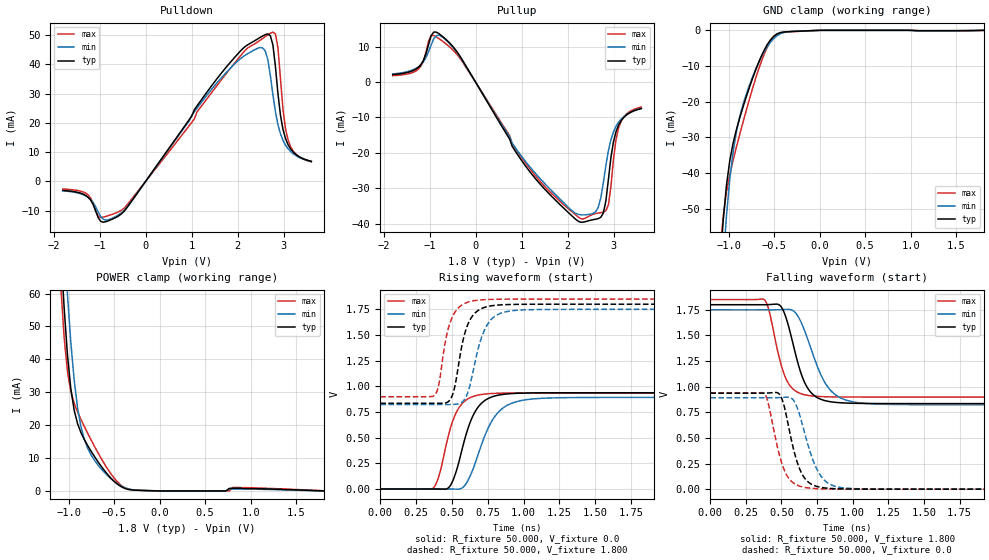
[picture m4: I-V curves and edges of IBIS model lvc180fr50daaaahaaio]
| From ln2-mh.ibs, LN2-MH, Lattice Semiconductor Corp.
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|   Model lvc180fr50daaaahaaio
[Model] lvc180fr50daaaahaaio
| Clamp models do not include dynamic input termination. Please refer to
| the lvc180axxxdaaaahaain model for input termination.
Model_type I/O
Polarity   Non-Inverting
Enable   Active-Low
Vinl =  0.630V
Vinh =  1.170V
Vmeas =  0.900V
Cref =  0.0F
Rref =  1.000M
Vref =  0.0V
C_comp   2.000pF   1.500pF   2.500pF
[Temperature Range]   25.000   0.125k   -40.000
[Voltage Range]   1.800V   1.750V   1.850V
[C Comp Corner]
C_comp   2.000pF   1.500pF   2.500pF
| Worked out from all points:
|   slope of the pulldown table from 0 to 0.27 V, typ, clamps not added: 44.9 ohm
|   slope of the pullup table from 0 to 0.27 V, typ, clamps not added: 45.5 ohm
|   GND clamp passes 1 mA (typ) near -0.47 V on its own axis
|   POWER clamp passes 1 mA (typ) near -0.40 V on its own axis
|   rising waveform, R_fixture 50.000, V_fixture 0.0: 20-80 % time 127ps typ, 160ps min, 110ps max; typ from 0 V to 0.938 V
|   rising waveform, R_fixture 50.000, V_fixture 1.800: 20-80 % time 87.8ps typ, 107ps min, 80.7ps max; typ from 0.835 V to 1.8 V
|   falling waveform, R_fixture 50.000, V_fixture 1.800: 20-80 % time 121ps typ, 162ps min, 101ps max; typ from 1.8 V to 0.835 V
|   falling waveform, R_fixture 50.000, V_fixture 0.0: 20-80 % time 102ps typ, 125ps min, 98.2ps max; typ from 0.937 V to 0 V
[Pulldown]
|Voltage   I(typ)   I(min)   I(max)
-1.8V     -3.079mA   -3.208mA   -2.604mA
-1.25V    -5.37mA    -5.445mA   -4.579mA
-975mV    -13.65mA   -11.99mA   -12.31mA
-480mV    -10.42mA   -10.07mA   -9.325mA
2.05V     44.35mA    41.79mA    42.66mA
2.545V    49.68mA    45.59mA    48.83mA
2.655V    50.36mA    41.57mA    50.03mA
2.765V    46.65mA    29.71mA    50.99mA
2.875V    29.99mA    19.42mA    45.69mA
2.93V     22.57mA    16.27mA    35.05mA
3.095V    12.53mA    11.14mA    14.19mA
3.6V      6.866mA    6.794mA    6.674mA
[Pullup]
|Voltage   I(typ)   I(min)   I(max)
-1.8V     2.133mA    2.309mA    1.821mA
-1.24V    4.215mA    4.333mA    3.727mA
-965mV    13.12mA    10.53mA    13.16mA
-745mV    13.21mA    12.97mA    11.84mA
1.125V    -24.42mA   -23.11mA   -23.58mA
2.28V     -39.63mA   -37.53mA   -38.61mA
2.665V    -38.63mA   -35.4mA    -37.04mA
2.83V     -33.63mA   -23.61mA   -36.38mA
2.885V    -27.55mA   -19.4mA    -34.71mA
2.995V    -16.89mA   -14.09mA   -21.87mA
3.105V    -12.18mA   -11.35mA   -12.99mA
3.6V      -7.446mA   -7.445mA   -7.067mA
[GND_clamp]
|Voltage   I(typ)   I(min)   I(max)
-1.8V     -571mA     -571.9mA   -573mA
-1.097V   -67.89mA   -81.9mA    -63.82mA
-1.06V    -53.86mA   -65.72mA   -52.69mA
-1.023V   -43.6mA    -52.29mA   -45.48mA
-986mV    -36.55mA   -41.78mA   -40.47mA
-949mV    -31.59mA   -33.97mA   -36.38mA
-912mV    -27.73mA   -28.25mA   -32.63mA
-838mV    -21.28mA   -20.51mA   -25.51mA
-616mV    -5.929mA   -6.39mA    -7.151mA
-468mV    -1.006mA   -1.514mA   -1.077mA
-24mV     -25.08uA   -21.99uA   -30.46uA
1.8V      -83.5nA    0A         -36.66uA
[POWER_clamp]
|Voltage   I(typ)   I(min)   I(max)
-1.789V   617.6mA    624.8mA    616.1mA
-1.086V   74.57mA    97.6mA     62.94mA
-1.049V   56.15mA    77.62mA    47.03mA
-1.012V   41.52mA    60.02mA    36.39mA
-975mV    31.15mA    45.29mA    30.27mA
-938mV    24.56mA    33.75mA    26.65mA
-901mV    20.5mA     25.36mA    24.04mA
-827mV    15.64mA    15.72mA    19.63mA
-679mV    8.958mA    7.957mA    11.71mA
-420mV    1.258mA    1.471mA    1.65mA
-13mV     8.76uA     8.311uA    10.26uA
1.8V      0A         0A         63.06uA
[Ramp]
| variable   typ   min   max
dV/dt_r   0.563/0.127n   0.536/0.160n   0.562/0.110n
dV/dt_f   0.579/0.121n   0.556/0.163n   0.571/0.101n
R_load = 50.000
[Rising Waveform]
R_fixture= 50.000
V_fixture= 0.0
V_fixture_min= 0.0
V_fixture_max= 0.0
|time   V(typ)   V(min)   V(max)
0s        2.404uV    12.25uV    1.1uV
369ps     71.87uV    58.48uV    8.909mV
411ps     -495.8uV   80.61uV    136.3mV
475ps     11.17mV    -333.7uV   519.2mV
598ps     527.8mV    50.69mV    865.8mV
666ps     763.7mV    267.7mV    909.3mV
764ps     888.9mV    626.7mV    928.9mV
914ps     929.1mV    833.7mV    935mV
1.244ns   937.1mV    888.8mV    936.2mV
10ns      937.5mV    892.5mV    936.2mV
[Rising Waveform]
R_fixture= 50.000
V_fixture= 1.800
V_fixture_min= 1.750
V_fixture_max= 1.850
|time   V(typ)   V(min)   V(max)
0s        834.8mV    822.8mV    898.8mV
382ps     834.7mV    822.8mV    918.4mV
407ps     834.5mV    822.8mV    1.008V
495ps     888mV      822.8mV    1.649V
568ps     1.387V     843.3mV    1.791V
613ps     1.61V      947.9mV    1.821V
656ps     1.707V     1.203V     1.834V
727ps     1.769V     1.548V     1.844V
826ps     1.792V     1.704V     1.848V
10ns      1.8V       1.75V      1.85V
[Falling Waveform]
R_fixture= 50.000
V_fixture= 1.800
V_fixture_min= 1.750
V_fixture_max= 1.850
|time   V(typ)   V(min)   V(max)
0s        1.8V       1.75V      1.85V
380ps     1.8V       1.75V      1.848V
491ps     1.79V      1.751V     1.247V
543ps     1.622V     1.755V     1.046V
611ps     1.252V     1.698V     947.8mV
671ps     1.017V     1.514V     918.8mV
749ps     895.4mV    1.208V     905.6mV
888ps     846mV      912mV      900.1mV
1.191ns   835.6mV    829.5mV    898.9mV
10ns      834.8mV    822.8mV    898.8mV
[Falling Waveform]
R_fixture= 50.000
V_fixture= 0.0
V_fixture_min= 0.0
V_fixture_max= 0.0
|time   V(typ)   V(min)   V(max)
0s        937.5mV    892.5mV    936.2mV
379ps     937.4mV    892.4mV    934.5mV
480ps     934.1mV    893.5mV    363.2mV
517ps     818.7mV    896.4mV    194.9mV
593ps     344.7mV    848.3mV    52.14mV
656ps     120.3mV    582.3mV    19.26mV
729ps     35.95mV    255.1mV    6.662mV
837ps     7.766mV    49.95mV    1.629mV
1.047ns   785.2uV    3.599mV    195.6uV
10ns      2.519uV    12.42uV    1.191uV
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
